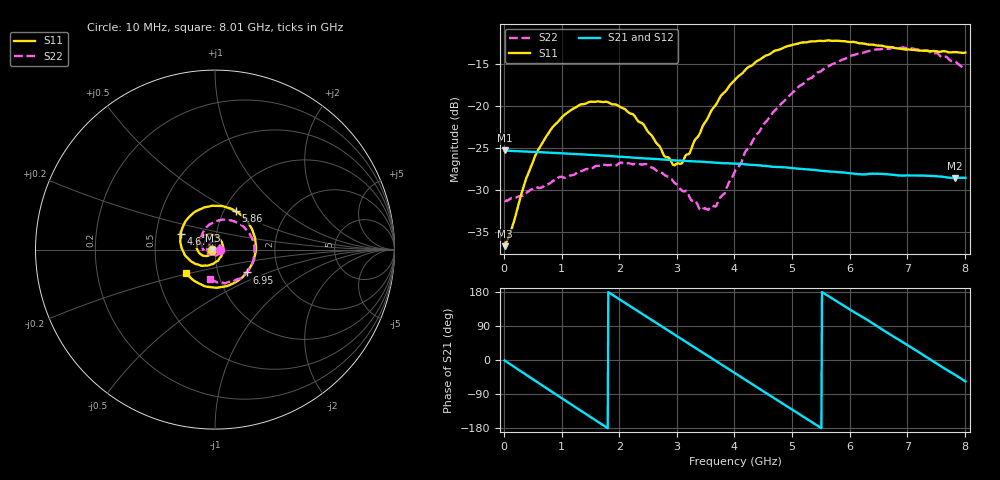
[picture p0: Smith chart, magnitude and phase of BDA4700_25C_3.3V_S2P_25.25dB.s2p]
!Agilent Technologies,E5071B,MY42404982,A.09.10
!Date: Mon Oct 20 18:13:41 2025
!Data & Calibration Information:
!Freq	S11:SOLT2(ON)	S21:SOLT2(ON)	S12:SOLT2(ON)	S22:SOLT2(ON)
# Hz S RI R 50
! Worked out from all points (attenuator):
!   801 points, 10 MHz to 8.01 GHz, reference 50 ohm
!   highest |S21| = -25.31 dB at 10 MHz (marker M1); lowest = -28.6 dB at 7.83 GHz (marker M2)
!   lowest |S11| = -36.7 dB at 10 MHz (marker M3), VSWR 1.03, Z = 48.6 - j0.126 ohm
!   |S11| at or under -10 dB: start of sweep to end of sweep
!   |S22| runs from -32.5 to -13.0 dB; largest |S21 - S12| = 0.00064
!   S11 on the Smith chart (normalised r, x): 10 MHz: 0.97, -0.00; 4.67 GHz: 0.67, +0.12; 5.86 GHz: 1.13, +0.52; 6.95 GHz: 1.37, -0.37; 8.01 GHz: 0.70, -0.19
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1e7  -0.0145 -0.0013  0.0542 -0.00115  0.0542 -0.00119  0.0271 -0.000797
1.4e8  -0.0159 -0.0102  0.0521 -0.0135  0.0521 -0.0134  0.0274 -0.00688
3.8e8  -0.0253 -0.0261  0.0417 -0.0334  0.0417 -0.0333  0.022 -0.0203
5.9e8  -0.0415 -0.0353  0.0267 -0.0457  0.0267 -0.0457  0.0139 -0.0295
1.01e9  -0.0826 -0.0241  -0.0105 -0.051  -0.0105 -0.0511  -0.0152 -0.0345
1.35e9  -0.1018 0.0111  -0.0366 -0.0361  -0.0366 -0.0361  -0.0365 -0.0183
2.07e9  -0.0457 0.0853  -0.0444 0.0221  -0.0444 0.0221  -0.0309 0.0334
2.68e9  0.0357 0.0463  -0.00331 0.048  -0.00344 0.0479  0.013 0.0383
2.93e9  0.0443 0.00562  0.0164 0.0445  0.0163 0.0444  0.0251 0.0254
3.06e9  0.0417 -0.0172  0.0257 0.0396  0.0253 0.0397  0.028 0.0155
3.43e9  -0.00112 -0.0729  0.0433 0.017  0.0432 0.017  0.0201 -0.0129
3.69e9  -0.0523 -0.0887  0.0456 -0.00291  0.0457 -0.00307  0.00143 -0.0253
4.01e9  -0.1239 -0.0711  0.0373 -0.0257  0.0372 -0.0257  -0.0311 -0.026
4.67e9  -0.192 0.0857  -0.00663 -0.0428  -0.00651 -0.0428  -0.0794 0.0453
5.35e9  -0.0551 0.2359  -0.0401 -0.0111  -0.04 -0.0113  -0.0158 0.1469
5.86e9  0.1151 0.2144  -0.0336 0.0218  -0.0335 0.0219  0.0977 0.1608
6.27e9  0.2087 0.107  -0.0129 0.0368  -0.0123 0.0369  0.183 0.1014
6.68e9  0.2209 -0.0405  0.0136 0.0365  0.0137 0.0366  0.2198 0.000145
6.95e9  0.176 -0.127  0.0274 0.027  0.0275 0.0268  0.2107 -0.0733
7.42e9  0.028 -0.2097  0.0382 -0.000299  0.0382 -0.000371  0.1233 -0.1647
7.83e9  -0.1138 -0.1758  0.0287 -0.0234  0.0287 -0.0235  0.0136 -0.1832
8.01e9  -0.1606 -0.1324  0.0205 -0.031  0.0206 -0.031  -0.0301 -0.1633
